{attribute 'call_after_init'}
FUNCTION_BLOCK FB_DS_IED_LD1_LLN0_DS3 EXTENDS FB_AcsiCommonDataSetClass
VAR
END_VAR

METHOD OnInit : BOOL
VAR
END_VAR
IF NOT DeleteAllMembers() THEN RETURN; END_IF
IF NOT AddMember(ipData:=fbIED.IEDLD1.XCBR1.Pos.stVal, eFc:=E_AcsiFc.ST_) THEN RETURN; END_IF
IF NOT AddMember(ipData:=fbIED.IEDLD1.XCBR1.Pos.q, eFc:=E_AcsiFc.ST_) THEN RETURN; END_IF
IF NOT AddMember(ipData:=fbIED.IEDLD1.XCBR1.Pos.t, eFc:=E_AcsiFc.ST_) THEN RETURN; END_IF
OnInit:= TRUE;
END_METHOD

END_FUNCTION_BLOCK
